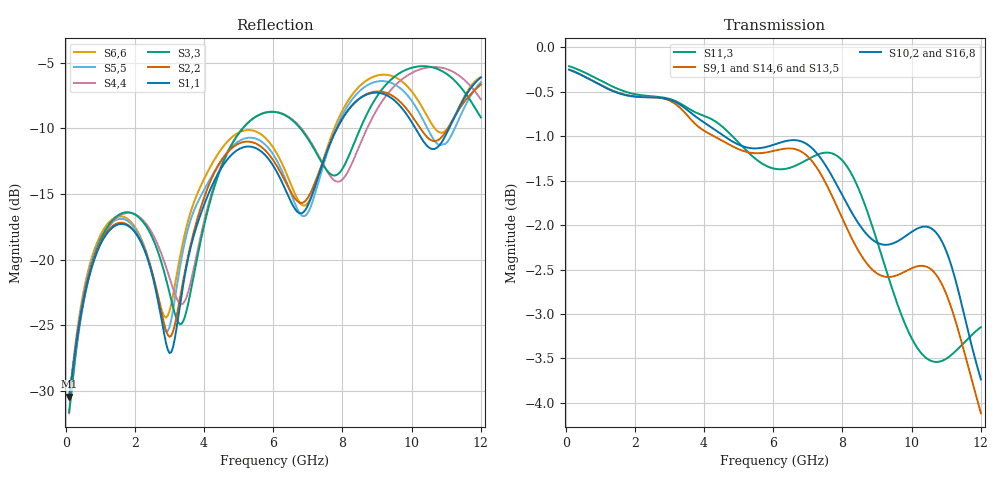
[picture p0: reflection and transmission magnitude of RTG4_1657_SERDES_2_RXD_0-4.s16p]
! RTG4 1657 S-parameter file
! Microsemi Corporation (c) 2019
!Initial ver: Jul 30, 2019
! Port::PIN_NAME::NET_NAME::S-parameter ports::PORT SIDE
! Port1:--:SERDES_2_RXD0_N_DIE::1::DIE
! Port2:--:SERDES_2_RXD0_P_DIE::2::DIE
! Port3:BA15:SERDES_2_RXD0_N_BGA::3::BGA
! Port4:AY15:SERDES_2_RXD0_P_BGA::4::BGA
! Port5:--:SERDES_2_RXD1_N_DIE::5::DIE
! Port6:--:SERDES_2_RXD1_P_DIE::6::DIE
! Port7:AW16:SERDES_2_RXD1_N_BGA::7::BGA
! Port8:AV16:SERDES_2_RXD1_P_BGA::8::BGA
! Port9:--:SERDES_2_RXD2_N_DIE::9::DIE
! Port10:--:SERDES_2_RXD2_P_DIE::10::DIE
! Port11:BA17:SERDES_2_RXD2_N_BGA::11::BGA
! Port12:AY17:SERDES_2_RXD2_P_BGA::12::BGA
! Port13:--:SERDES_2_RXD3_N_DIE::13::DIE
! Port14:--:SERDES_2_RXD3_P_DIE::14::DIE
! Port15:BA19:SERDES_2_RXD3_N_BGA::15::BGA
! Port16:AY19:SERDES_2_RXD3_P_BGA::16::BGA
!TouchstoneFormatFlag = 1
! GNDNET
! NETSLIST
! User Comments:
! Touchstone file exported from HFSS 2018.2.0
!  File:  C:/Users/LSI_SIM_01/Desktop/Microsemi_190710/YBD197_150320_NETCHANGE_SERDES_2_RXD.aedt
!  Generated:  1:11:18 ??  7 12, 2019
!  Design:  HFSSModel1
!  Project:  YBD197_150320_NETCHANGE_SERDES_2_RXD
!  Setup:  Setup1
!  Solution:  Sweep
! Terminal data exported
! Port[1] = SERDES_2_RXD0_N_DIE
! Port[2] = SERDES_2_RXD0_P_DIE
! Port[3] = SERDES_2_RXD1_N_DIE
! Port[4] = SERDES_2_RXD1_P_DIE
! Port[5] = SERDES_2_RXD2_N_DIE
! Port[6] = SERDES_2_RXD2_P_DIE
! Port[7] = SERDES_2_RXD3_N_DIE
! Port[8] = SERDES_2_RXD3_P_DIE
! Port[9] = SERDES_2_RXD0_N_BGA
! Port[10] = SERDES_2_RXD0_P_BGA
! Port[11] = SERDES_2_RXD1_N_BGA
! Port[12] = SERDES_2_RXD1_P_BGA
! Port[13] = SERDES_2_RXD2_N_BGA
! Port[14] = SERDES_2_RXD2_P_BGA
! Port[15] = SERDES_2_RXD3_N_BGA
! Port[16] = SERDES_2_RXD3_P_BGA
# GHZ S DB R 50.000000
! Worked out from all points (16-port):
!   239 points, 100 MHz to 12 GHz, reference 50 ohm
!   strongest paths, dB at 100 MHz, 3.05 GHz, 6.05 GHz, 9.05 GHz, 12 GHz:
!     S10,2: -0.2, -0.6, -1.1, -2.2, -3.7
!     S9,1: -0.3, -0.6, -1.2, -2.6, -4.1
!     S14,6: -0.2, -0.6, -1.2, -2.6, -4.4
!     S11,3: -0.2, -0.6, -1.4, -2.2, -3.1
!     S16,8: -0.3, -0.6, -1.2, -2.4, -3.8
!     S13,5: -0.2, -0.7, -1.3, -2.9, -4.2
!   lowest |S11| = -30.4 dB at 100 MHz (marker M1), VSWR 1.06, Z = 52.7 - j1.52 ohm
!   |S11| at or under -10 dB: start of sweep to 7.84 GHz; 10.11 GHz to 11.08 GHz (972.6 MHz wide, 9.18 % of centre)
